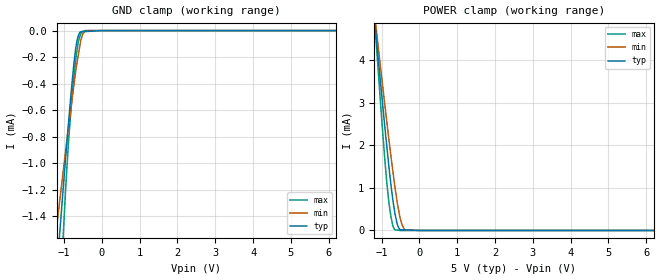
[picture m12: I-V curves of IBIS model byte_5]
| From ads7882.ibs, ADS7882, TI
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|   byte_5 Model
[Model]   byte_5
Model_type   Input
Vinl = 0.8
Vinh = 4
|   typ   min   max
|   (nom PVT)   (Fast PVT)   (slow PVT)
|C_comp from frequency sweep method (F=1.5MHz)
|Average
C_comp   2.470e-12   2.396e-12   2.543e-12
|C_comp from LC tank measurement(L=1nH)
|Resonant Frequency(Hz)   3.600e+09   3.640e+09   3.530e+09
|C_comp   1.956e-12   1.914e-12   2.035e-12
| Where nom  PVT is Nominal Process,  5V,  25C
|   Fast PVT is Strong Process,   5.25V,  -40C
|   Slow PVT is Weak Process,   4.75V,  85C
[Model Spec]
Vinh   4   3.75   4.25
[Voltage Range]   5   4.75   5.25
|Ambient Temperature   25   85   -40
|Junction Temperature
[Temperature Range]   25   85   -40
[Power Clamp Reference]   5   4.75   5.25
[GND Clamp Reference]   0   0   0
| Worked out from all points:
|   GND clamp passes 1 mA (typ) near -0.97 V on its own axis
|   POWER clamp passes 1 mA (typ) near -0.74 V on its own axis
[GND Clamp]
|   Voltage   I(typ)   I(min)   I(max)
-5V       -16.63mA   -11.21mA   -29.39mA
-1.246V   -2.011mA   -1.606mA   -2.946mA
-1.125V   -1.565mA   -1.31mA    -2.168mA
-1.02V    -1.176mA   -1.053mA   -1.529mA
-884mV    -699.7uA   -731.4uA   -845.7uA
-789.5mV  -393.3uA   -521.8uA   -498.9uA
-685mV    -121uA     -290uA     -203.1uA
-621.5mV  -39.54uA   -180.7uA   -79.94uA
-570mV    -9.736uA   -93.95uA   -34.5uA
-511.2mV  -8.733uA   -29.91uA   -5.026uA
-373.5mV  -6.38uA    0A         0A
10V       0A         0A         0A
[POWER Clamp]
|   Voltage   I(typ)   I(min)   I(max)
-5V       42.59mA    36.62mA    54.91mA
-1.246V   5.536mA    5.572mA    5.704mA
-1.029V   3.485mA    3.846mA    3.011mA
-905mV    2.354mA    2.887mA    1.569mA
-810.5mV  1.537mA    2.17mA     688uA
-705.5mV  745.9uA    1.422mA    124uA
-653mV    436.4uA    1.061mA    17.98uA
-585mV    147.7uA    654uA      9.353uA
-506.5mV  19.36uA    280.8uA    0A
-454.2mV  17.36uA    117.5uA    0A
-373.5mV  14.27uA    14.02uA    0A
10V       0A         0A         0A
